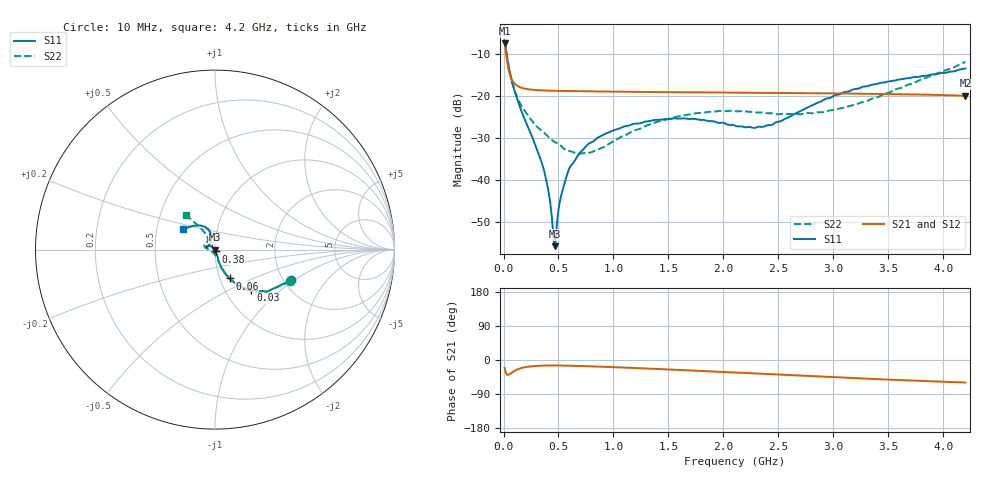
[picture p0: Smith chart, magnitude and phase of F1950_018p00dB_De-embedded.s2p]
! Integrated Device Technology
! Corporate Headquarters
! 6024 Silver Creek Valley Road
! San Jose, CA 95138  USA
! Phone:  1-408-284-8200
! Toll Free:  1-800-223-1366
! Webpage:  http://www.idt.com/
! Timing and RF Division
! 515 Groton Road, Suite 102
! Westford, MA 01886-6024
! Device:  F1950
! Description: 7-bit 0.25 dB Digital Step Attenuator
! Frequency:  150.0 -  4000.00 MHz
! Package:  4x4 mm Thin QFN Plastic Package: 24 pin
! Ports:  2 RF, 12 DC
!  Pin  1  = D0
!  Pin  2  = VDD
!  Pin  3  = Vmode
!  Pin  4  = GND
!  Pin  5  = RF1  =  Port 1
!  Pin  6  = GND
!  Pin  7  = GND
!  Pin  8  = GND
!  Pin  9  = GND
!  Pin 10  = GND
!  Pin 11  = GND
!  Pin 12  = GND
!  Pin 13  = GND
!  Pin 14  = RF2  =  Port 2
!  Pin 15  = GND
!  Pin 16  = LE
!  Pin 17  = CLK
!  Pin 18  = DATE
!  Pin 19  = D6
!  Pin 20  = D5
!  Pin 21  = D4
!  Pin 22  = D3
!  Pin 23  = D2
!  Pin 24  = D1
! State:  72
! Atten State:  18.00 dB
! Voltage:  +5.00 Volts
! Current:  Not Measured mA
! Data:  The device was measured on a the F195X evaluation board which has
!  individual transmission lines to the RF pins.  Data was collected
!  using a calibrated network analyzer.  The evaluation board was
!  de-embedded using a TRL calibration technique.
!  The reference plane is the edge of the package pin.
! Misc:  Board 2019
!  Action Tracker AT0250
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# GHz S dB R 50
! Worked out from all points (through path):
!   420 points, 10 MHz to 4.2 GHz, reference 50 ohm
!   highest |S21| = -7.50 dB at 10 MHz (marker M1); lowest = -20.0 dB at 4.2 GHz (marker M2)
!   group delay of S21, straight-line fit = 31.1 ps
!   lowest |S11| = -55.7 dB at 470 MHz (marker M3), VSWR 1.00, Z = 49.8 - j0.0237 ohm
!   |S11| at or under -10 dB: 27.8 MHz to end of sweep
!   |S22| runs from -33.8 to -6.8 dB; largest |S21 - S12| = 0.00017
!   S11 on the Smith chart (normalised r, x): 10 MHz: 2.18, -0.94; 30 MHz: 1.31, -0.65; 60 MHz: 1.11, -0.37; 380 MHz: 1.01, -0.02; 4.2 GHz: 0.68, +0.17
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0.01  -6.84 -22.1  -7.50 -21.1  -7.50 -21.1  -6.84 -22.8
0.03  -10.40 -48.7  -11.36 -38.3  -11.36 -38.3  -10.36 -49.3
0.06  -14.87 -63.0  -15.11 -36.6  -15.11 -36.6  -14.61 -63.2
0.11  -19.57 -70.8  -17.34 -27.1  -17.34 -27.1  -19.41 -69.3
0.16  -23.43 -72.0  -18.06 -21.5  -18.06 -21.5  -22.24 -73.3
0.32  -33.81 -71.3  -18.66 -15.3  -18.66 -15.3  -27.71 -80.2
0.38  -39.03 -70.2  -18.73 -14.7  -18.73 -14.7  -29.02 -82.4
0.42  -44.46 -79.1  -18.77 -14.5  -18.77 -14.5  -30.03 -84.5
0.45  -52.04 -101.3  -18.79 -14.5  -18.79 -14.5  -30.70 -88.3
0.47  -55.73 -171.6  -18.80 -14.5  -18.80 -14.5  -31.02 -91.2
0.52  -44.20 142.2  -18.83 -14.6  -18.83 -14.6  -31.82 -95.1
0.58  -38.55 135.9  -18.86 -14.9  -18.86 -14.9  -33.06 -104.9
0.71  -33.12 138.5  -18.90 -15.9  -18.90 -15.9  -33.67 -126.2
0.95  -28.75 146.7  -18.99 -18.3  -18.99 -18.3  -31.57 -163.1
1.41  -25.70 163.8  -19.11 -23.8  -19.10 -23.8  -26.07 170.1
1.73  -25.46 169.4  -19.17 -27.9  -19.17 -27.9  -24.20 161.3
2.11  -27.13 159.4  -19.25 -33.1  -19.25 -33.1  -23.66 152.4
2.43  -26.95 127.5  -19.31 -37.2  -19.31 -37.3  -24.15 143.4
2.81  -22.23 105.9  -19.38 -42.6  -19.38 -42.6  -24.14 129.4
3.1  -19.08 107.5  -19.45 -46.6  -19.45 -46.6  -22.80 123.3
3.51  -16.53 117.9  -19.57 -51.9  -19.57 -52.0  -19.20 121.5
4.2  -13.48 146.4  -19.98 -59.3  -19.97 -59.4  -11.96 130.3
